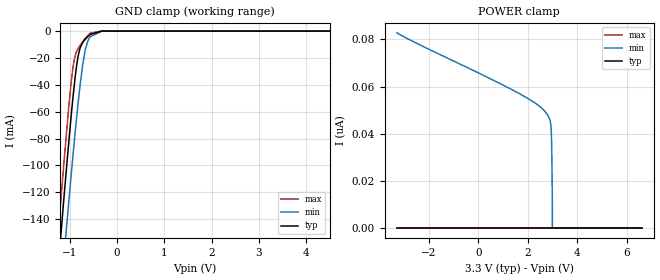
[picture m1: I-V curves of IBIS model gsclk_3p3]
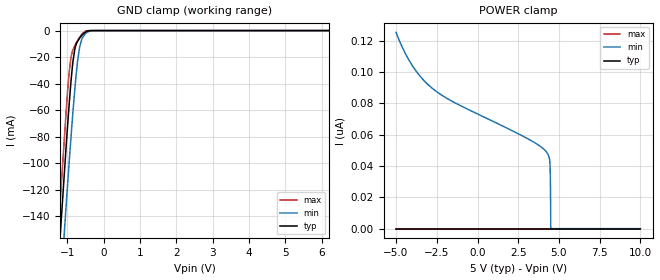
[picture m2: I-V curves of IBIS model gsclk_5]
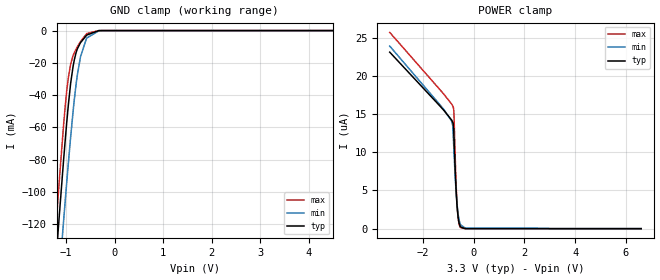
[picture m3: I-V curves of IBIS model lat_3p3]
|Texas Instruments Incorporated
| 48 channels, 16bit PWM LED driver with dot correction
| Marketing part#   Digital Voltage Range   Package-type   #pins
| TLC5955DCAR   3.0V-5.5V   HTSSOP   56
| TLC5955DCA   3.0V-5.5V   HTSSOP   56
| TLC5955RTQR   3.0V-5.5V   QFN   56
| TLC5955RTQT   3.0V-5.5V   QFN   56
[IBIS Ver]   4.1
[File name]   tlc5955.ibs
[File Rev]   1.0
[Date]   2/17/2014
[Source]
| Texas Instruments Incorporated.
| Analog-eLab Design Center, HPA
| 12500 TI Blvd
| Dallas, TX -75243
[Notes]   Revision History:
| Rev 1.0: 2/17/2014
| - Initial version of the model
| - Model generated from simulations in TISPICE
| - Model matched to SPICE simulation
| - C_comp although listed in numerical order of value are
|   obtained from varying PVT conditions. For PVT conditions for
|   each specific value refer the buffer description under
|   respective [Model]. IBIS model user is responsible for using
|   appropriate C_comp to simulate for Signal Integrity.
[Disclaimer]
| This model is designed as an aid for customers of Texas Instruments.
| TI and its licensors and suppliers make no warranties, either expressed
| or implied, with respect to this  model, including the warranties of
| merchantability or fitness for a particular purpose. The model is
| provided solely on an "as is" basis. The entire risk as to its quality
| and performance is with the customer.
[Copyright]
(C) Copyright 2014 Texas Instruments Incorporated.All rights reserved.
|   TLC5955DCA
[Component]   TLC5955DCA
[Manufacturer]   TI
[Package]   |56 HTSSOP  -  DCA package
|   typ   min   max
R_pkg   0.01   0.008   0.12
L_pkg   1.0nH   0.8nH   1.2nH
C_pkg   0.2pF   0.16pF   0.24pF
[Pin]  signal_name   model_name   R_pin   L_pin   C_pin
1   SIN   SIN   NA   NA   NA
2   SCLK   SCLK   NA   NA   NA
3   LAT   LAT   NA   NA   NA
4   OUTB4   NC   NA   NA   NA
5   OUTR4   NC   NA   NA   NA
6   OUTG4   NC   NA   NA   NA
7   OUTB0   NC   NA   NA   NA
8   OUTR0   NC   NA   NA   NA
9   OUTG0   NC   NA   NA   NA
10   OUTB5   NC   NA   NA   NA
11   OUTR5   NC   NA   NA   NA
12   OUTG5   NC   NA   NA   NA
13   OUTB1   NC   NA   NA   NA
14   OUTR1   NC   NA   NA   NA
15   OUTG1   NC   NA   NA   NA
16   OUTB2   NC   NA   NA   NA
17   OUTR2   NC   NA   NA   NA
18   OUTG2   NC   NA   NA   NA
19   OUTB6   NC   NA   NA   NA
20   OUTR6   NC   NA   NA   NA
21   OUTG6   NC   NA   NA   NA
22   OUTB3   NC   NA   NA   NA
23   OUTR3   NC   NA   NA   NA
24   OUTG3   NC   NA   NA   NA
25   OUTB7   NC   NA   NA   NA
26   OUTR7   NC   NA   NA   NA
27   OUTG7   NC   NA   NA   NA
28   SOUT   SOUT   NA   NA   NA
29   GND   GND   NA   NA   NA
30   OUTG11   NC   NA   NA   NA
31   OUTR11   NC   NA   NA   NA
32   OUTB11   NC   NA   NA   NA
33   OUTG15   NC   NA   NA   NA
34   OUTR15   NC   NA   NA   NA
35   OUTB15   NC   NA   NA   NA
36   OUTG10   NC   NA   NA   NA
37   OUTR10   NC   NA   NA   NA
38   OUTB10   NC   NA   NA   NA
39   OUTG14   NC   NA   NA   NA
40   OUTR14   NC   NA   NA   NA
41   OUTB14   NC   NA   NA   NA
42   OUTG13   NC   NA   NA   NA
43   OUTR13   NC   NA   NA   NA
44   OUTB13   NC   NA   NA   NA
45   OUTG9   NC   NA   NA   NA
46   OUTR9   NC   NA   NA   NA
47   OUTB9   NC   NA   NA   NA
48   OUTG12   NC   NA   NA   NA
49   OUTR12   NC   NA   NA   NA
50   OUTB12   NC   NA   NA   NA
51   OUTG8   NC   NA   NA   NA
52   OUTR8   NC   NA   NA   NA
53   OUTB8   NC   NA   NA   NA
54   VCC   POWER   NA   NA   NA
55   GSCLK   GSCLK   NA   NA   NA
56   GND   GND   NA   NA   NA
|   TLC5955RTQ
[Component]   TLC5955RTQ
[Manufacturer]   TI
[Package]   |56 QFN   -  RTQ package
|   typ   min   max
R_pkg   0.01   0.008   0.12
L_pkg   1.0nH   0.8nH   1.2nH
C_pkg   0.2pF   0.16pF   0.24pF
[Pin]  signal_name   model_name   R_pin   L_pin   C_pin
1   OUTB3   NC   NA   NA   NA
2   OUTR3   NC   NA   NA   NA
3   OUTG3   NC   NA   NA   NA
4   OUTB7   NC   NA   NA   NA
5   OUTR7   NC   NA   NA   NA
6   OUTG7   NC   NA   NA   NA
7   SOUT   SOUT   NA   NA   NA
8   GND   GND   NA   NA   NA
9   OUTG11   NC   NA   NA   NA
10   OUTR11   NC   NA   NA   NA
11   OUTB11   NC   NA   NA   NA
12   OUTG15   NC   NA   NA   NA
13   OUTR15   NC   NA   NA   NA
14   OUTB15   NC   NA   NA   NA
15   OUTG10   NC   NA   NA   NA
16   OUTR10   NC   NA   NA   NA
17   OUTB10   NC   NA   NA   NA
18   OUTG14   NC   NA   NA   NA
19   OUTR14   NC   NA   NA   NA
20   OUTB14   NC   NA   NA   NA
21   OUTG13   NC   NA   NA   NA
22   OUTR13   NC   NA   NA   NA
23   OUTB13   NC   NA   NA   NA
24   OUTG9   NC   NA   NA   NA
25   OUTR9   NC   NA   NA   NA
26   OUTB9   NC   NA   NA   NA
27   OUTG12   NC   NA   NA   NA
28   OUTR12   NC   NA   NA   NA
29   OUTB12   NC   NA   NA   NA
30   OUTG8   NC   NA   NA   NA
31   OUTR8   NC   NA   NA   NA
32   OUTB8   NC   NA   NA   NA
33   VCC   POWER   NA   NA   NA
34   GSCLK   GSCLK   NA   NA   NA
35   GND   GND   NA   NA   NA
36   SIN   SIN   NA   NA   NA
37   SCLK   SCLK   NA   NA   NA
38   LAT   LAT   NA   NA   NA
39   OUTB4   NC   NA   NA   NA
40   OUTR4   NC   NA   NA   NA
41   OUTG4   NC   NA   NA   NA
42   OUTB0   NC   NA   NA   NA
43   OUTR0   NC   NA   NA   NA
44   OUTG0   NC   NA   NA   NA
45   OUTB5   NC   NA   NA   NA
46   OUTR5   NC   NA   NA   NA
47   OUTG5   NC   NA   NA   NA
48   OUTB1   NC   NA   NA   NA
49   OUTR1   NC   NA   NA   NA
50   OUTG1   NC   NA   NA   NA
51   OUTB2   NC   NA   NA   NA
52   OUTR2   NC   NA   NA   NA
53   OUTG2   NC   NA   NA   NA
54   OUTB6   NC   NA   NA   NA
55   OUTR6   NC   NA   NA   NA
56   OUTG6   NC   NA   NA   NA
|   Model Selectors
[Model Selector] GSCLK
gsclk_3p3   3.3V  digital input
gsclk_5   5.0V  digital input
[Model Selector] LAT
lat_3p3   3.3V  digital input
lat_5   5.0V  digital input
[Model Selector] SCLK
sclk_3p3   3.3V  digital input
sclk_5   5.0V  digital input
[Model Selector] SIN
sin_3p3   3.3V  digital input
sin_5   5.0V  digital input
[Model Selector] SOUT
sout_3p3   3.3V  digital output
sout_5   5.0V  digital output
| Models and submodels in the file (10): gsclk_3p3 (Input), gsclk_5 (Input), lat_3p3 (Input), lat_5 (Input), sclk_3p3 (Input), sclk_5 (Input), sin_3p3 (Input), sin_5 (Input), sout_3p3 (Output), sout_5 (Output)
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|   gsclk_3p3 Model
[Model]   gsclk_3p3
Model_type   Input
Vinl = 0.99
Vinh = 2.31
|   typ   min   max
|   (nom PVT)   (fast PVT)   (slow PVT)
C_comp   1.424e-12   1.397e-12   1.472e-12
[Model spec]
|subparameter
Vinl   0.99   0.9   1.08
Vinh   2.31   2.1   2.52
| Where nom  PVT is Nominal Process, 3.3V, 27C
|   Fast PVT is Strong Process,  3.6V, -40C
|   Slow PVT is Weak Process,   3V, 125C
[Voltage Range]   3.3   3   3.6
|Junction Temperature
[Temperature Range]   27   125   -40
[Power Clamp Reference]   3.3   3   3.6
[GND Clamp Reference]   0   0   0
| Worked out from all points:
|   GND clamp passes 1 mA (typ) near -0.42 V on its own axis
[GND Clamp]
|   Voltage   I(typ)   I(min)   I(max)
-3.3V     -1.128A    -1.136A    -1.132A
-1.3V     -198.5mA   -240.6mA   -174.3mA
-1.14V    -129.9mA   -173.9mA   -103.8mA
-1.119V   -121.2mA   -165.4mA   -94.88mA
-1.025V   -83.05mA   -127.6mA   -56.75mA
-954mV    -56.23mA   -100.1mA   -32.35mA
-898.8mV  -37.45mA   -79.39mA   -19.85mA
-825mV    -18.54mA   -53.45mA   -12.95mA
-675mV    -6.126mA   -14.1mA    -5.384mA
-564mV    -2.468mA   -4.153mA   -1.544mA
-246mV    -1.523uA   -28.85uA   -70.53nA
6.6V      0A         0A         0A
[POWER Clamp]
|   Voltage   I(typ)   I(min)   I(max)
-3.3V     0A         82.73nA    0A
1.605V    0A         57.3nA     0A
2.403V    0A         52.19nA    0A
2.739V    0A         48.87nA    0A
2.895V    0A         45.66nA    0A
2.943V    0A         41.92nA    0A
2.961V    0A         36.38nA    0A
2.976V    0A         26.6nA     0A
2.985V    0A         17.73nA    0A
2.991V    0A         10.45nA    0A
2.993V    0A         0A         0A
6.6V      0A         0A         0A
|   gsclk_5 Model
[Model]   gsclk_5
Model_type   Input
Vinl = 1.5
Vinh = 3.5
|   typ   min   max
|   (nom PVT)   (fast PVT)   (slow PVT)
C_comp   1.384e-12   1.346e-12   1.437e-12
[Model spec]
|subparameter
Vinl   1.5   1.35   1.65
Vinh   3.5   3.15   3.85
| Where nom  PVT is Nominal Process, 5V, 27C
|   Fast PVT is Strong Process,  5.5V, -40C
|   Slow PVT is Weak Process,   4.5V, 125C
[Voltage Range]   5   4.5   5.5
|Junction Temperature
[Temperature Range]   27   125   -40
[Power Clamp Reference]   5   4.5   5.5
[GND Clamp Reference]   0   0   0
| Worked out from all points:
|   GND clamp passes 1 mA (typ) near -0.50 V on its own axis
[GND Clamp]
|   Voltage   I(typ)   I(min)   I(max)
-5V       -1.943A    -1.925A    -1.966A
-1.252V   -177.4mA   -220.1mA   -152.5mA
-1.19V    -151mA     -194.5mA   -125.4mA
-1.026V   -83.72mA   -128.2mA   -57.4mA
-952mV    -55.51mA   -99.29mA   -31.76mA
-915mV    -42.68mA   -85.37mA   -22.7mA
-846.5mV  -23.03mA   -60.75mA   -14.37mA
-750mV    -9.753mA   -30.53mA   -8.868mA
-662mV    -5.629mA   -12.14mA   -4.842mA
-594.5mV  -3.34mA    -5.658mA   -2.395mA
-500mV    -1.061mA   -2.203mA   -419.1uA
10V       0A         0A         0A
[POWER Clamp]
|   Voltage   I(typ)   I(min)   I(max)
-5V       0A         125.3nA    0A
-3.992V   0A         104nA      0A
-2.785V   0A         89.71nA    0A
3.095V    0A         57.35nA    0A
4.212V    0A         49.22nA    0A
4.364V    0A         46.53nA    0A
4.441V    0A         42.18nA    0A
4.459V    0A         37.18nA    0A
4.473V    0A         29.3nA     0A
4.49V     0A         10.96nA    0A
4.495V    0A         0A         0A
10V       0A         0A         0A
|   lat_3p3 Model
[Model]   lat_3p3
Model_type   Input
Vinl = 0.99
Vinh = 2.31
|   typ   min   max
|   (nom PVT)   (fast PVT)   (slow PVT)
C_comp   1.546e-12   1.501e-12   1.609e-12
[Model spec]
|subparameter
Vinl   0.99   0.9   1.08
Vinh   2.31   2.1   2.52
| Where nom  PVT is Nominal Process, 3.3V, 27C
|   Fast PVT is Strong Process,  3.6V, -40C
|   Slow PVT is Weak Process,   3V, 125C
[Voltage Range]   3.3   3   3.6
|Junction Temperature
[Temperature Range]   27   125   -40
[Power Clamp Reference]   3.3   3   3.6
[GND Clamp Reference]   0   0   0
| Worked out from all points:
|   GND clamp passes 1 mA (typ) near -0.42 V on its own axis
[GND Clamp]
|   Voltage   I(typ)   I(min)   I(max)
-3.3V     -1.076A    -1.077A    -1.087A
-1.33V    -191.3mA   -226.2mA   -172.2mA
-1.169V   -124.9mA   -161.9mA   -103.5mA
-1.057V   -81.28mA   -119mA     -59.54mA
-960mV    -47.23mA   -83.44mA   -29.95mA
-907.5mV  -32.39mA   -65.47mA   -20.68mA
-859.2mV  -22.28mA   -50.19mA   -15.54mA
-795mV    -13.47mA   -32.84mA   -11.38mA
-708mV    -7.591mA   -16.51mA   -6.931mA
-573mV    -2.734mA   -4.552mA   -1.795mA
-246mV    -1.528uA   -28.93uA   -71.11nA
6.6V      0A         0A         0A
[POWER Clamp]
|   Voltage   I(typ)   I(min)   I(max)
-3.3V     23.11uA    23.91uA    25.7uA
-1.169V   15.49uA    15.59uA    17.61uA
-861.3mV  14.22uA    14.06uA    16.31uA
-822mV    13.97uA    13.51uA    16.08uA
-801.9mV  13.75uA    12.41uA    15.93uA
-772.8mV  12.2uA     10.29uA    15.19uA
-700.8mV  6.038uA    5.585uA    7.144uA
-650.1mV  3.045uA    3.235uA    3.188uA
-607.2mV  1.516uA    1.9uA      1.369uA
-510mV    225.5nA    494.3nA    131.3nA
-240.9mV  0A         70.22nA    0A
6.6V      0A         0A         0A
